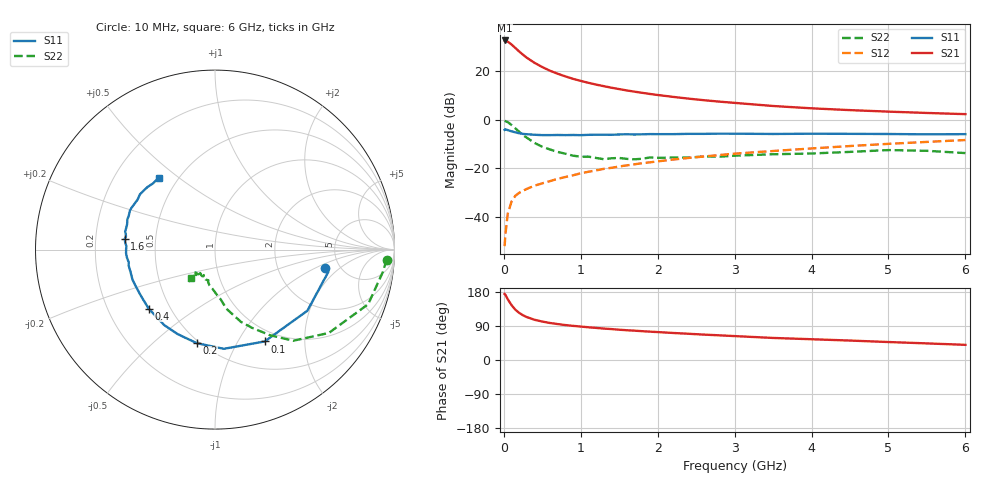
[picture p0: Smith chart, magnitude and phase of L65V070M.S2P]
!  INFINEON TECHNOLOGIES Small Signal Semiconductors
! BFR380L3 , Si-NPN RF-Transistor in TSLP-3-1
!  Vce=5 V,  Ic=70 mA
! Common Emitter S-Parameters:  07. March 2005
#  GHz  S  MA  R  50
! f  S11  S21  S12  S22
! GHz  Mag  Ang  Mag  Ang  Mag  Ang  Mag  Ang
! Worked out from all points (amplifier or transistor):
!   36 points, 10 MHz to 6 GHz, reference 50 ohm
!   highest |S21| = 32.8 dB at 10 MHz (marker M1)
!   |S21| within 3 dB of that: start of sweep to 146.4 MHz
!   unconditionally stable (mu >= 1): 1.373 GHz to 4.795 GHz
!   at 250 MHz: K = 0.51, MSG = 28.0 dB, |S12| = -29.2 dB
!   at 1.4 GHz: K = 1.00, MAG = 16.1 dB, |S12| = -19.7 dB
!   at 6 GHz: K = 0.97, MSG = 5.3 dB, |S12| = -8.3 dB
!   S11 on the Smith chart (normalised r, x): 10 MHz: 3.86, -1.27; 100 MHz: 0.84, -1.30; 200 MHz: 0.48, -0.70; 400 MHz: 0.38, -0.33; 1.6 GHz: 0.33, +0.05; 6 GHz: 0.39, +0.43
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0.01  0.6233 -9.3  43.46 174.2  0.0025 73.0  0.9582 -3.3
0.02  0.6435 -11.1  43.08 172.2  0.0043 88.8  0.9429 -7.7
0.05  0.6172 -33.5  41.21 160.6  0.0115 74.6  0.9061 -19.6
0.1  0.5818 -61.6  35.86 144.8  0.0208 67.1  0.7862 -36.2
0.15  0.5549 -84.9  30.41 132.7  0.0274 59.6  0.6697 -49.3
0.2  0.5311 -101.0  25.69 124.2  0.0315 58.1  0.5691 -57.1
0.25  0.5146 -113.9  22.04 118.0  0.0347 55.3  0.4819 -64.7
0.3  0.507 -123.9  19.07 113.1  0.038 55.0  0.4283 -70.2
0.4  0.4945 -138.3  15 106.1  0.0442 55.6  0.3355 -79.1
0.5  0.4866 -147.9  12.28 101.4  0.0493 58.0  0.2799 -83.4
0.6  0.4865 -155.0  10.32 97.7  0.0548 59.4  0.2463 -88.5
0.7  0.4894 -160.0  8.961 94.8  0.0611 61.3  0.2189 -93.7
0.9  0.4894 -169.6  7.027 90.1  0.0724 63.6  0.1832 -102.2
1.1  0.4926 -174.8  5.817 86.3  0.0854 65.1  0.175 -107.1
1.3  0.4953 179.5  4.963 82.9  0.0981 66.2  0.155 -113.8
1.6  0.5065 173.1  4.051 78.5  0.1159 66.7  0.1575 -122.1
2.2  0.5096 163.9  2.988 71.3  0.1525 67.5  0.1673 -124.3
2.8  0.5214 155.4  2.386 65.1  0.1888 67.3  0.1746 -130.9
3.5  0.5135 147.1  1.938 58.2  0.229 65.0  0.1962 -129.8
4.5  0.5166 141.1  1.593 51.3  0.2898 63.4  0.2194 -129.5
5.5  0.5051 133.0  1.392 43.8  0.3524 59.8  0.2309 -129.2
6  0.5095 128.0  1.316 40.0  0.3855 57.6  0.2073 -130.5
